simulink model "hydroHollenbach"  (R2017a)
settings: Solver=VariableStepAuto  StartTime=0.0  StopTime=10.0  RelTol=1e-3

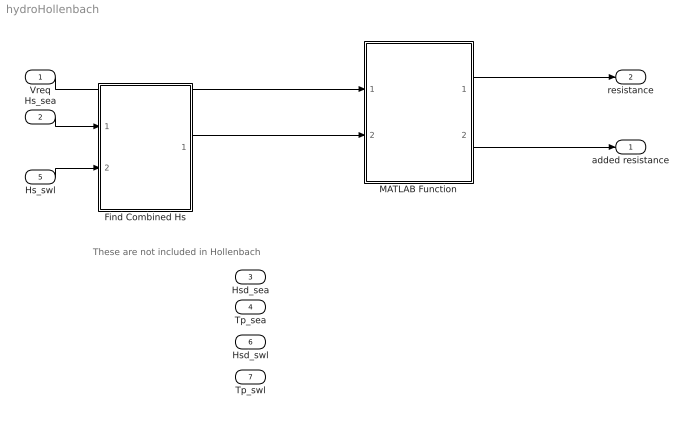
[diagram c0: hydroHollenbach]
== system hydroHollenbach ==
  note: These are not included in Hollenbach
  Vreq : Inport
  Hs_sea : Inport  Port=2
  Hsd_sea : Inport  Port=3
  Tp_sea : Inport  Port=4
  Hs_swl : Inport  Port=5
  Hsd_swl : Inport  Port=6
  Tp_swl : Inport  Port=7
  Find Combined Hs : MATLAB Function  TreatAsAtomicUnit=on
  MATLAB Function : MATLAB Function  TreatAsAtomicUnit=on
  added resistance : Outport
  resistance : Outport  Port=2
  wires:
  Vreq/1 -> MATLAB Function/1(Vreq)
  Hs_sea/1 -> Find Combined Hs/1(Hs_Sea)
  MATLAB Function/1(R) -> resistance/1
  MATLAB Function/2(Raw) -> added resistance/1
  Hs_swl/1 -> Find Combined Hs/2(Hs_Swell)
  Find Combined Hs/1(Hs_combined) -> MATLAB Function/2(Hst)

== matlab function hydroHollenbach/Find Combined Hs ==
function Hs_combined = Combine_Hs(Hs_Sea,Hs_Swell)


Hs_combined=((Hs_Sea^2)+(Hs_Swell^2))^0.5;
end

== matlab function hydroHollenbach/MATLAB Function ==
% Function that uses Hollenbachs method, and Kreitner to find resistance%
% Author:   Peter Tenfjord and Martin Bakke 
% Date:     01.06.2017
% Reference is made to (Steen and Minsaas, 2013)


function [R, Raw] = hollenb(Vreq, Hst, num)

%%%%%%%%%%%%%%%%%%%%%%%%%%%%%%%%%%%%%%%%%%%%%%%%%%%%%%%%%%%
%            Hollenbach.m
%%%%%%%%%%%%%%%%%%%%%%%%%%%%%%%%%%%%%%%%%%%%%%%%%%%%%%%%%%%

%output: R [N] and Raw [N]


% Ship velocities in m/s
 Vs = Vreq*0.5144;



%constants
rho = 1025;
gravk = 9.81;   %Gravity
nu = 1.1395E-6; % viscosity

%ship particulars from vessel info
Los = num(1); 
L = num(2); 
Lwl = num(3); 
B=num(4);  
CB=num(8); 
k=num(9); 

    T = num(6); 
    TA = num(6);
    TF = num(7); 
    Dp = num(10);
    NRud = num(11); 
    NBrac = num(12); 
    NBoss = num(13); 
    NThr = num(14);
    S = num(15); 
    
Lfn=Los;
%%%%%%%%%%%%%%%%%%%%%%%%%%%%%%%%%%%%%%%%%%%%%%%%%%%%%%%%%%%
% Constants from Hollenbachs paper: 
%%%%%%%%%%%%%%%%%%%%%%%%%%%%%%%%%%%%%%%%%%%%%%%%%%%%%%%%%%%

% 'Mean' resistance coefficients
   a = num(16:25);  	
%a1 means a(1) and so on
   b = [num(26:28); 	%b12 means b(1,2)
	    num(29:31);
        num(32:34)];
    
   d = num(36:38);
   e = num(39:40);
   f = num(41:43);
   g = num(44:46);


	% Froude's number
	Fn = Vs/sqrt(gravk*Lfn);			
	Fnkrit = d*[1 CB CB^2]';
    
	c1 = Fn/Fnkrit;
	c1_min = 0;
	
	Rns = Vs*L/nu;						% Reynold's number for ship
	CFs = 0.075/(log10(Rns)-2)^2;			% ITTC friction line for ship				

	% Calculation of C_R for given ship 
	% Mean value
	
	CRFnkrit = max(1.0,(Fn/Fnkrit)^c1);
	
	kL = e(1)*L^(e(2));
	

    
	% There is an error in the hollenbach paper and in Minsaas' 2003 textbook, which
	% is corrected in this formula by dividing by 10
	CRstandard = [1 CB CB^2]*(b*[1 Fn Fn^2]')/10;
	
	CR_hollenbach = CRstandard*CRFnkrit*kL*prod([T/B B/L Los/Lwl Lwl/L (1+(TA-TF)/L) ...
			Dp/TA (1+NRud) (1+NBrac) (1+NBoss) (1+NThr)].^a);
	
	CR = CR_hollenbach*B*T/S;   			% Resistance coefficient, scaled for wetted surface
	C_Ts = CFs + CR;				        % Total resistance coeff. ship 
	R_T_mean = C_Ts*rho/2*Vs^2*S;			% Total resistance to the ship
	
	%%%%%%%%%%%%%%%%%%%%%%%%%%%%%%%%%%%%%%%%%%%%%%%%%%%%%%%%%%%
	% When accounting for form factor, roughness and correlation coef.,  as given by Minsaas
	Rnm = 6*sqrt(6/L)*10^6/1.1395*Vs;		% Reynold's number for model
	CFm = 0.075/(log10(Rnm)-2)^2;			% ITTC friction line for model
	dCF = (110.31*(150*Vs/0.514)^0.21 - 403.33)*CFs^2; % Increase in friction due to roughness
	CA = -0.228*10^(-3);					% Correlation coefficient
	CR_2 = CR_hollenbach*B*T/S - k*CFm;		% Resistance coefficient 
	C_Ts_2 = (1+k)*(CFs + dCF) + CR_2 + CA;	% Total resistance coeff. ship 
	R_T_mean_2 = C_Ts_2*rho/2*Vs^2*S;		% Total resistance to the ship

	%%%%%%%%%%%%%%%%%%%%%%%%%%%%%%%%%%%%%%%%%%%%%%%%%%%%%%%%%%%%%%%%%%%%%%%%
	
R = max(R_T_mean_2,R_T_mean); %N

% estimate of the added resistance due to waves, from Kreitner (ITTC 2005)
% Should only be used on waves up to two meters in height. 
% If waves are larger, then a Raw is taken as a conservative 20% of R

if Hst<=2
    Raw=(0.64*Hst^2*num(4)^2*num(8)*rho*gravk/num(3)); %N
else
    Raw=0.20*R;
end
    
    
    
end
